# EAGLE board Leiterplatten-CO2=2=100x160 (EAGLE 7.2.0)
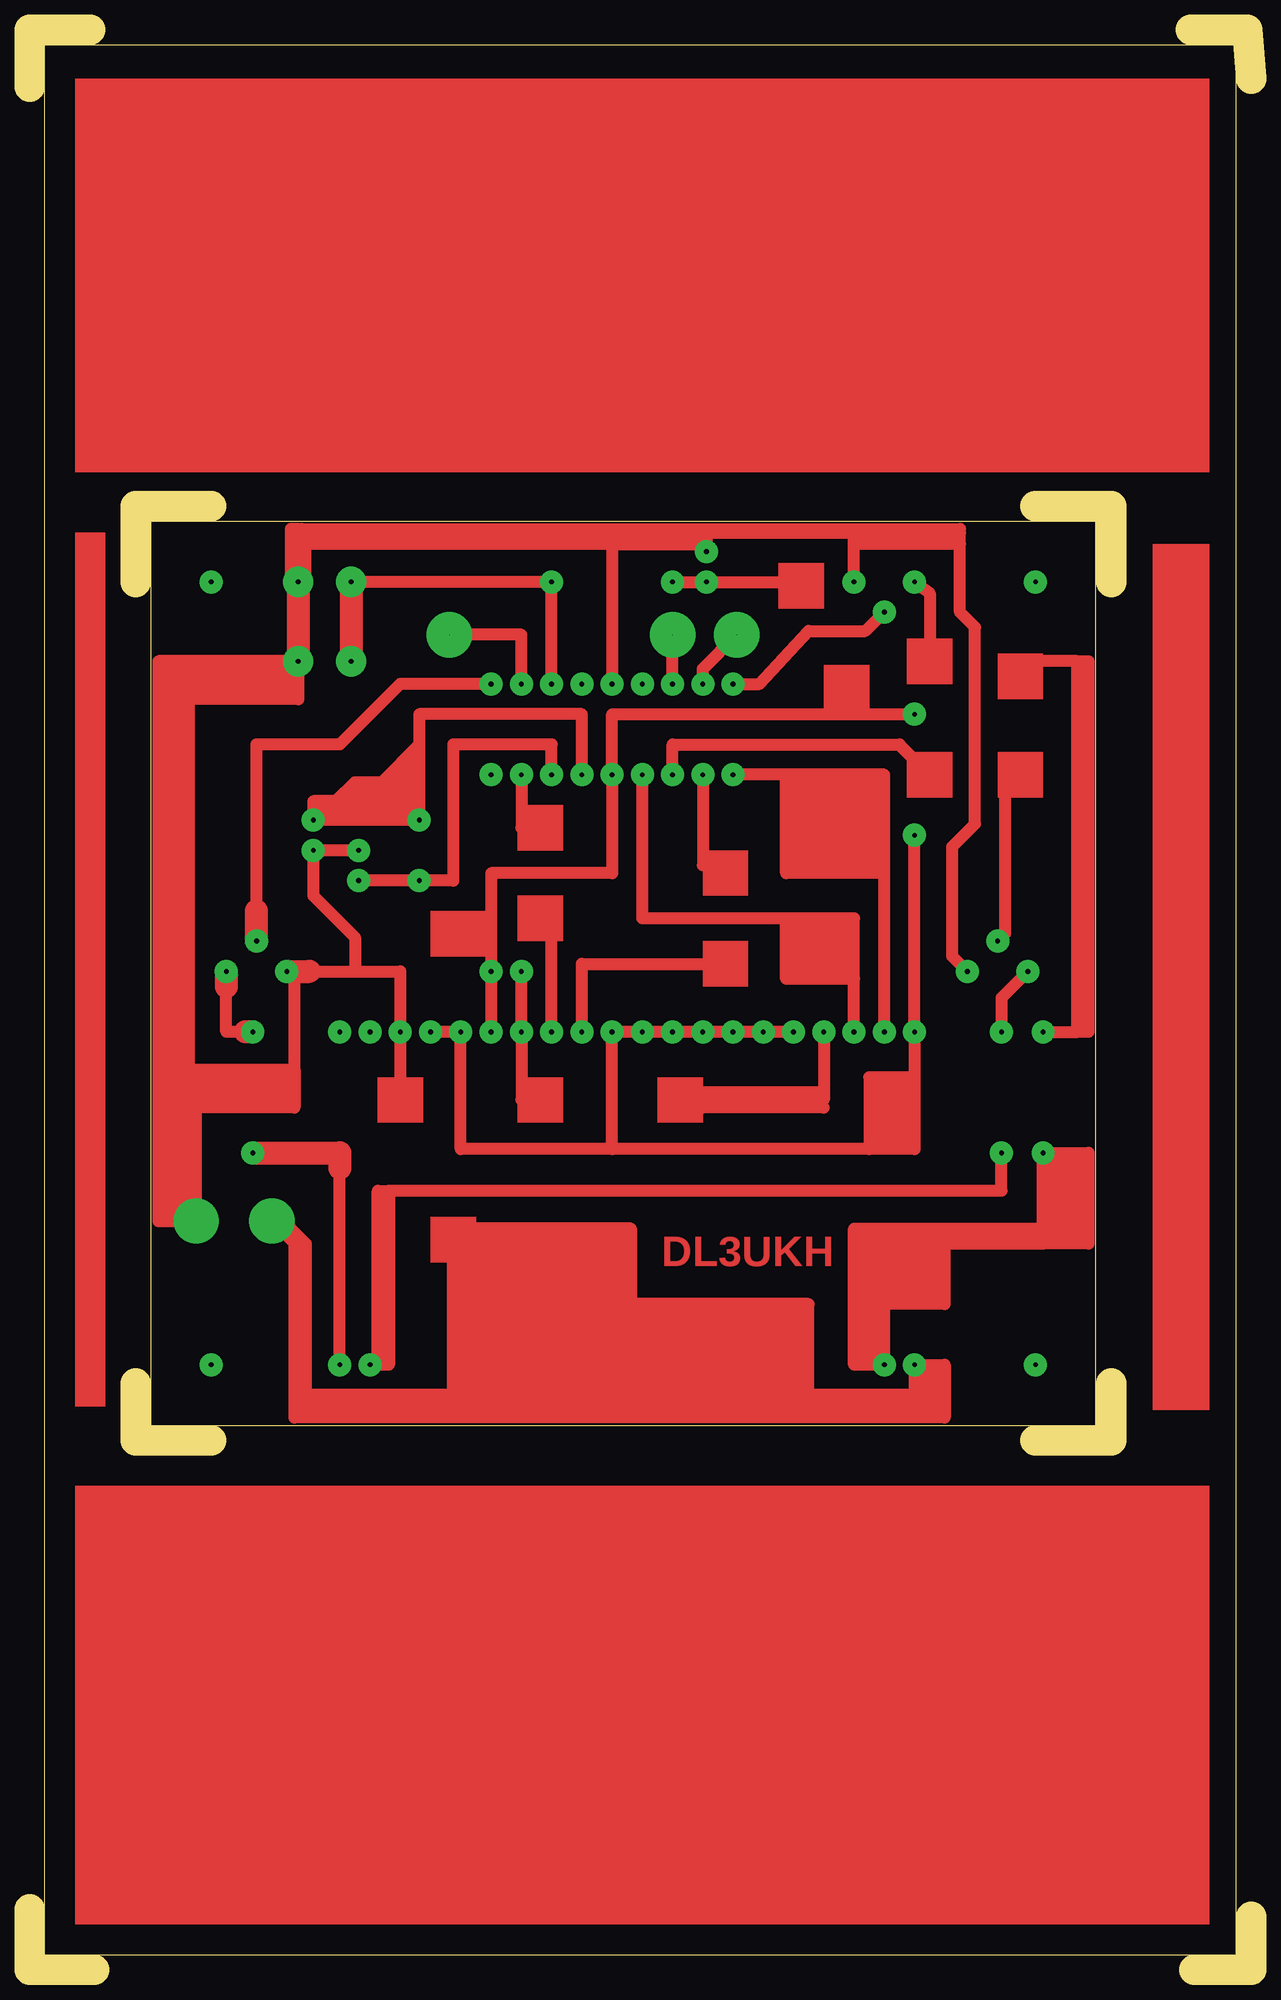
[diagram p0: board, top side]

Size 102.55 x 162.88 mm. Coordinates in mm from the lower left corner, seen from the top.
Outline: 5.4,0 0.32,0
Outline: 0,0 0,5.08
Outline: 97.79,0 102.55,0 102.55,4.45
Outline: 5.08,162.88 0,162.88 0,158.12
Outline: 102.55,158.75 102.23,162.88 97.47,162.88
Outline: 8.89,116.52 8.89,122.87 15.24,122.87
Outline: 8.89,49.21 8.89,44.45 15.24,44.45
Outline: 84.45,44.45 90.8,44.45 90.8,49.21
Outline: 90.8,116.52 90.8,122.87 84.45,122.87
Outline: 1.27,1.27 101.28,1.27 101.28,161.61 1.27,161.61 1.27,1.27
Outline: 10.16,121.6 10.16,45.72 89.53,45.72 89.53,121.6 10.16,121.6
Copper layers (1*16): Top 0.035mm / dielectric 1.5mm / Bottom 0.035mm
Design rules "default": minimum track width 10mil, minimum drill 24mil, track to track 8mil, track to pad 8mil, pad to pad 8mil, via to via 8mil, smd to smd 8mil, copper to edge 40mil, drill to drill 8mil, minimum pad ring 10mil, minimum via ring 8mil, stop-mask expansion 4mil, vias tented up to drill 0mil, thermal gap 10mil

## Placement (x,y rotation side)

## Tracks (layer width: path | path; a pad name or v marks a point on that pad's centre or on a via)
S$1  (via drill 0.4 pad 1.93)
  Top 1.016: v38.74,78.74 v38.74,83.82 38.74,86.99 | 38.74,86.99 38.74,92.08 48.9,92.08 v48.9,100.33 48.9,105.41 74.3,105.41 | 38.74,86.99 35.56,86.99
S$2  (via drill 0.4 pad 1.93)
  other vias: 59.05,78.74
S$3  (via drill 0.4 pad 1.93)
  Top 1.016: v53.98,100.33 53.98,102.87 73.02,102.87 75.56,100.33
S$4  (via drill 0.4 pad 1.93)
  Top 1.016: v56.52,100.33 56.52,92.71 58.42,92.71
S$5  (via drill 0.4 pad 1.93)
  Top 1.016: v41.28,100.33 41.28,95.88 42.86,95.88
S$6  (via drill 0.01 pad 3.81, 0.4 pad 1.93, 0.4 pad 2.54)
  Top 1.016: v78.74,83.82 77.47,85.09 77.47,94.3 79.38,96.2 79.38,112.71 78.1,113.98 78.1,119.7 | 78.1,119.7 78.1,120.65 69.21,120.65 | 13.33,109.85 v22.54,109.85 22.54,106.68 13.33,106.68 | 13.33,109.85 13.33,106.68 | 13.33,106.68 13.33,75.56 | 13.33,75.56 13.97,75.56 | 13.97,75.56 22.22,75.56 | v22.54,116.52 22.54,119.7 | 22.54,119.7 22.54,120.65 | 22.54,120.65 22.86,120.65 | 22.86,120.65 48.9,120.65 | 48.9,120.65 48.9,119.7 | 48.9,119.7 v48.9,107.95 | 48.9,120.65 56.83,120.65 | 56.83,120.65 69.21,120.65 | v69.21,116.52 69.21,120.65 | 22.22,75.56 22.22,83.19 v21.59,83.82 | v27.62,93.98 v23.81,93.98 23.81,90.17 27.3,86.68 27.3,83.82 | 23.5,83.82 27.3,83.82 | 27.3,83.82 31.11,83.82 v31.11,78.74 31.11,73.34 | 56.83,120.65 56.83,119.7 | 56.83,119.7 v56.83,119.06 | 13.97,75.56 v13.97,62.87 10.79,62.87 10.79,75.56 | 13.33,75.56 10.79,75.56 | 22.22,75.56 22.22,72.39 13.65,72.39 | 13.33,109.85 10.79,109.85 10.79,75.56 | 22.54,120.65 22.54,120.97 | 22.54,120.97 22.86,120.97 | 22.86,120.97 78.1,120.97 | 48.9,119.7 22.54,119.7 | 48.9,119.7 56.83,119.7 | 78.1,119.7 69.53,119.7 | 22.86,120.65 22.86,120.97 | 22.54,120.97 21.91,120.97 21.91,116.52
  Top 1.93: v22.54,116.52 v22.54,109.85 | v21.59,83.82 23.5,83.82
S$7  (via drill 0.4 pad 1.93)
  Top 1.016: v41.28,107.95 41.28,112.08 35.24,112.08
S$8  (via drill 0.4 pad 1.93)
  other vias: 84.45,50.8
S$9  (via drill 0.4 pad 1.93)
  other vias: 84.45,116.52
S$10  (via drill 0.4 pad 1.93)
  Top 1.016: v53.98,116.52 64.77,116.52
S$11  (via drill 0.4 pad 1.93)
  other vias: 56.52,78.74
S$12  (via drill 0.4 pad 1.93)
  Top 1.016: 30.16,65.41 81.6,65.41 v81.6,68.58 | 30.16,65.41 30.16,50.8 29.21,50.8 | 29.21,50.8 v28.57,50.8 | 29.21,50.8 29.21,65.41 30.16,65.41
S$13  (via drill 0.4 pad 1.93)
  other vias: 74.3,105.41
S$14  (via drill 0.4 pad 1.93)
  Top 1.016: v46.36,78.74 46.36,84.45 58.42,84.45
S$15  (via drill 0.4 pad 1.93)
  Top 1.016: v66.67,78.74 66.67,73.66 | 66.67,73.66 66.67,73.02 55.56,73.02 | 66.67,73.66 55.88,73.66
S$16  (via drill 0.4 pad 1.93)
  Top 1.016: v74.3,116.52 75.56,115.57 75.56,109.85
S$17  (via drill 0.4 pad 1.93)
  Top 1.016: v81.28,86.36 81.91,86.99 81.91,99.69
S$18  (via drill 0.4 pad 1.93)
  Top 1.016: 77.15,60.96 85.09,60.96 | 71.75,62.23 69.21,62.23 69.21,50.8 v71.75,50.8 71.75,55.88 | 71.75,62.23 76.83,62.23 | 76.83,62.23 85.09,62.23 | 85.09,62.23 v85.09,68.58 88.9,68.58 88.9,60.96 85.09,60.96 | 71.75,55.88 71.75,62.23 | 76.83,61.6 76.83,55.88 71.75,55.88 | 76.83,61.6 76.83,62.23 | 85.09,60.96 85.09,61.6 | 85.09,62.23 85.09,61.6 | 85.09,61.6 76.83,61.6
S$19  (via drill 0.4 pad 1.93)
  Top 1.016: v26.04,50.8 26.04,67.31
  Top 1.93: v18.73,68.58 26.04,68.58 26.04,67.31
S$20  (via drill 0.4 pad 1.93)
  Top 1.016: v43.82,100.33 43.82,102.87 35.56,102.87 35.56,91.44 v32.7,91.44 v27.62,91.44
S$21  (via drill 0.4 pad 1.93)
  Top 1.016: v53.98,107.95 53.98,111.76
S$22  (via drill 0.4 pad 1.93)
  other vias: 38.74,100.33
S$23  (via drill 0.4 pad 1.93)
  Top 1.016: v74.3,95.25 v74.3,78.74 74.3,74.93 | 74.3,74.93 74.3,68.9 70.48,68.9 | 70.48,68.9 48.9,68.9 | v64.14,78.74 v61.6,78.74 v53.98,78.74 v48.9,78.74 48.9,68.9 | v33.66,78.74 v36.2,78.74 36.2,68.9 48.9,68.9 | 74.3,74.93 70.48,74.93 70.48,68.9
S$24  (via drill 0.4 pad 1.93)
  Top 1.016: v43.82,78.74 43.82,87.31
S$25  (via drill 0.4 pad 1.93)
  other vias: 28.57,78.74
S$26  (via drill 0.4 pad 1.93)
  other vias: 26.04,78.74
S$27  (via drill 0.4 pad 1.93)
  Top 1.016: v85.09,78.74 87.95,78.74 | 87.95,78.74 87.95,109.85 | 87.95,109.85 81.91,109.85 | 87.95,109.85 88.9,109.85 88.9,78.74 87.95,78.74
S$28  (via drill 0.01 pad 3.81, 0.4 pad 1.93)
  Top 1.016: 35.88,62.23 50.48,62.23 50.48,55.88 | 74.3,48.26 v74.3,50.8 76.83,50.8 76.83,46.99 | 74.3,48.26 74.3,46.99 | 74.3,46.99 35.56,46.99 | 35.56,46.99 35.56,55.88 | 35.56,55.88 35.56,61.28 | 35.56,46.99 22.22,46.99 | 22.22,46.99 22.22,48.26 | 22.22,48.26 22.22,60.96 | 22.22,60.96 v20.32,62.87 | 76.83,46.99 74.3,46.99 | 74.3,48.26 22.22,48.26 | 76.83,46.99 76.83,46.36 22.22,46.36 22.22,46.99 | 65.41,47.62 65.41,55.88 50.48,55.88 | 50.48,55.88 35.56,55.88 | 22.22,60.96 23.18,60.96 | 23.18,60.96 23.18,47.62 | 23.18,60.96 20.64,63.5
S$29  (via drill 0.4 pad 1.93)
  other vias: 15.24,50.8
S$30  (via drill 0.4 pad 1.93)
  Top 1.016: 19.05,88.9 19.05,102.87 26.04,102.87 31.11,107.95 v38.74,107.95
  Top 1.93: v19.05,86.36 19.05,88.9
S$31  (via drill 0.4 pad 1.93)
  Top 1.016: v59.05,107.95 61.28,107.95 65.41,112.39 70.17,112.39 v71.75,113.98
S$32  (via drill 0.4 pad 1.93)
  other vias: 51.44,107.95
S$33  (via drill 0.4 pad 1.93)
  Top 1.016: 18.1,78.74 16.51,78.74 16.51,82.55
  Top 1.93: v16.51,83.82 16.51,82.55 | v18.73,78.74 18.1,78.74
S$34  (via drill 0.4 pad 1.93)
  other vias: 15.24,116.52
S$35  (via drill 0.4 pad 1.93)
  Top 1.016: v41.28,83.82 v41.28,78.74 41.28,73.02
S$36
  Top 1.016: 66.67,72.39 56.52,72.39
S$37  (via drill 0.01 pad 3.81)
  other vias: 53.98,112.08
S$38  (via drill 0.01 pad 3.81, 0.4 pad 1.93)
  Top 1.016: v71.75,78.74 71.75,92.08 | 71.75,92.08 71.75,100.33 63.5,100.33 | 63.5,100.33 v59.05,100.33 | v56.52,107.95 56.52,109.22 v59.37,112.08 59.69,112.39 | 71.75,92.08 63.5,92.08 63.5,100.33
S$39  (via drill 0.01 pad 3.81)
  other vias: 35.24,112.08
S$41  (via drill 0.4 pad 1.93)
  other vias: 46.36,107.95
S$42  (via drill 0.4 pad 1.93)
  Top 1.016: v83.82,83.82 81.6,81.6 v81.6,78.74
S$43
  Top 1.016: 23.18,116.52 23.18,120.02
S$44  (via drill 0.4 pad 1.93)
  Top 1.016: v69.21,78.74 69.21,83.19 | 69.21,83.19 69.21,88.27 63.5,88.27 | 63.5,88.27 51.44,88.27 v51.44,100.33 | 69.21,83.19 63.5,83.19 63.5,88.27
S$45  (via drill 0.4 pad 1.93, 0.4 pad 2.54)
  Top 1.016: v43.82,107.95 v43.82,116.52 v26.99,116.52
  Top 1.93: v26.99,116.52 v26.99,109.85
S$46  (via drill 0.4 pad 1.93)
  other vias: 56.83,116.52
S$48  (via drill 0.4 pad 1.93)
  other vias: 51.44,78.74
S$57  (via drill 0.4 pad 1.93)
  Top 1.016: v46.36,100.33 46.36,105.41 32.7,105.41 32.7,102.87 | 32.7,102.87 v32.7,96.52 v23.81,96.52 23.81,98.11 25.72,98.11 27.3,99.69 29.53,99.69 32.7,102.87
(copper drawn outside any net)
  shapes: Top area x39

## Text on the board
Top: DL3UKH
